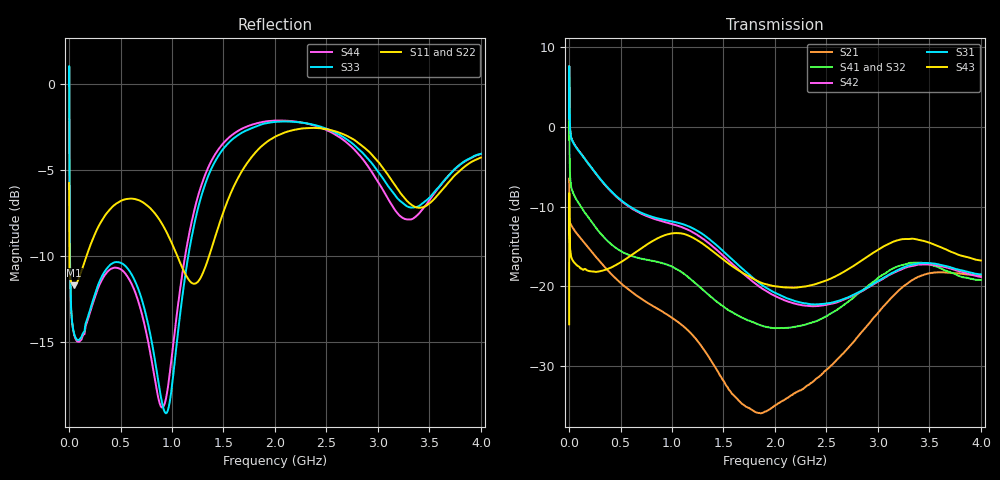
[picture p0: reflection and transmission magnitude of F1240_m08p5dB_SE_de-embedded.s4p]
! Integrated Device Technology
! Corporate Headquarters
! 6024 Silver Creek Valley Road
! San Jose, CA 95138  USA
! Phone:  1-408-284-8200
! Toll Free:  1-800-223-1366
! Webpage:  http://www.idt.com/
! Timing and RF Division
! 515 Groton Road, Suite 102
! Westford, MA 01886-6024
! Device:  F1240
! Description: Dual Intermediate Frequency Digital Variable Gain Amplifier
! Frequency:  10.0 -  500.00 MHz
! Package:  5x5 mm QFN Plastic Package: 32 pin
! Ports:  8 RF, 20 DC
!  Pin  1  = GA3 / Data  Pin 17  = RF OUT_B+
!  Pin  2  = GA4 / CLK  Pin 18  = RF OUT_B-
!  Pin  3  = GA5  Pin 19  = STBY_B
!  Pin  4  = VMODE  Pin 20  = Ground
!  Pin  5  = No Connect  Pin 21  = Ground
!  Pin  6  = GB5  Pin 22  = STB_A
!  Pin  7  = GB4  Pin 23  = RF OUT_A-  = Port 4
!  Pin  8  = GB3  Pin 24  = RF OUT_A+  = Port 3
!  Pin  9  = GB2  Pin 25  = GA0
!  Pin 10  = GB1  Pin 26  = ISET_A
!  Pin 11  = RF IN_B+  Pin 27  = VCC
!  Pin 12  = RF IN_B-  Pin 28  = Ground
!  Pin 13  = Ground  Pin 29  = RF IN_A-  = Port 2
!  Pin 14  = VCC  Pin 30  = RF IN_A+  = Port 1
!  Pin 15  = ISET_B  Pin 31  = GA1
!  Pin 16  = GB0  Pin 32  = GA2 / CSb
! Gain  = +19.5 dB
! State  = 1
! Voltage  = +5.00 V
! Current  = 85.292 mA (one channel only)
! Temperture  =  +25 C
! Test Date  =  2017-10-18
! Board  =  EB4031
! Data:  The device was measured on a custom evaluation board which has
!  individual transmission lines to the RF pins.  Data was collected
!  using a calibrated network analyzer.  The evaluation board was
!  de-embedded using Automatic Fixture Removal.
!  The reference plane is the edge of the package pin.
!  Only Channel A was measured.
!  This data is in single-ended operation.  If your needs are balanced
!  or differential S-parameters then this file needs to be used a
!  linear simulator.
! File Date:  2017-11-10  MJV
! Note:
!  Integrated Device Technology supplies this data as a sample of measured
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# Hz S dB R 100
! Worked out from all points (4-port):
!   410 points, 500 kHz to 4 GHz, reference 100 ohm
!   strongest paths, dB at 500 kHz, 930 MHz, 1.96 GHz, 2.98 GHz, 4 GHz:
!     S43: -24.8, -13.6, -19.9, -15.6, -16.8
!     S31: 1.1, -11.7, -20.6, -19.5, -18.5
!     S42: 1.1, -11.9, -21.0, -19.6, -18.8
!     S41: -1.6, -17.2, -25.2, -19.2, -19.2
!     S32: -1.5, -17.4, -25.0, -19.4, -19.5
!     S21: -6.5, -23.4, -35.3, -23.7, -18.7
!   lowest |S11| = -11.7 dB at 50 MHz (marker M1), VSWR 1.70, Z = 144 - j47.4 ohm
!   |S11| at or under -10 dB: 2.932 MHz to 169.2 MHz (166.3 MHz wide, 193 % of centre); 1.052 GHz to 1.36 GHz (307.8 MHz wide, 25.5 % of centre)
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500000  -5.74 -5.6  -6.48 -5.8  -31.70 77.4  -34.23 76.4
        -6.50 -5.8  -5.73 -5.6  -34.18 75.2  -31.70 78.5
        1.05 -111.1  -1.53 -113.0  -0.09 -0.1  -24.79 -38.8
        -1.55 -111.9  1.05 -110.0  -24.78 -38.9  -0.10 2.2
3500000  -10.43 -20.4  -11.42 -18.5  -24.78 4.3  -29.55 -10.8
         -11.42 -18.6  -10.44 -20.6  -29.52 -11.0  -24.77 4.5
         3.75 156.0  -1.03 140.9  -3.97 -83.4  -10.58 175.7
         -1.06 141.1  3.75 156.2  -10.59 175.7  -4.02 -83.4
5e7  -11.70 -36.2  -12.94 -22.4  -26.20 -17.6  -32.46 -20.7
     -12.95 -22.4  -11.67 -36.6  -32.48 -20.5  -26.17 -17.6
     -2.21 151.6  -8.61 142.8  -14.52 -164.5  -17.06 152.2
     -8.60 142.8  -2.16 151.5  -17.03 152.1  -14.59 -165.1
5e8  -6.79 -143.0  -19.58 -123.8  -29.96 -100.8  -37.22 -93.1
     -19.57 -123.6  -6.75 -143.7  -37.33 -90.8  -30.26 -100.7
     -9.15 29.5  -15.68 -16.7  -10.38 -173.4  -17.09 13.9
     -15.57 -18.1  -9.23 27.9  -17.01 13.6  -10.75 -174.0
2.06e9  -2.89 -179.0  -34.34 60.2  -33.37 -20.1  -35.62 0.7
        -34.48 60.8  -2.80 -179.5  -36.21 7.2  -34.83 -13.7
        -21.18 62.4  -25.14 -5.2  -2.17 175.0  -20.34 32.8
        -25.24 -12.5  -21.58 65.2  -20.11 33.9  -2.11 171.9
2.92e9  -3.96 100.7  -24.61 -24.9  -28.86 -153.5  -31.19 -139.7
        -24.59 -25.0  -3.75 101.5  -31.73 -126.6  -30.23 -145.0
        -19.99 -69.5  -20.02 -149.5  -4.45 92.5  -16.88 -93.7
        -19.78 -161.3  -20.05 -66.1  -16.10 -91.7  -4.92 85.1
4e9  -4.26 -127.3  -18.66 122.2  -27.33 -21.9  -28.32 -6.9
     -18.66 122.2  -4.02 -125.9  -28.93 6.4  -29.11 -11.5
     -18.52 54.9  -19.46 -39.1  -4.05 -133.0  -18.13 61.7
     -19.21 -53.3  -18.84 61.1  -16.77 55.4  -4.05 -142.9
